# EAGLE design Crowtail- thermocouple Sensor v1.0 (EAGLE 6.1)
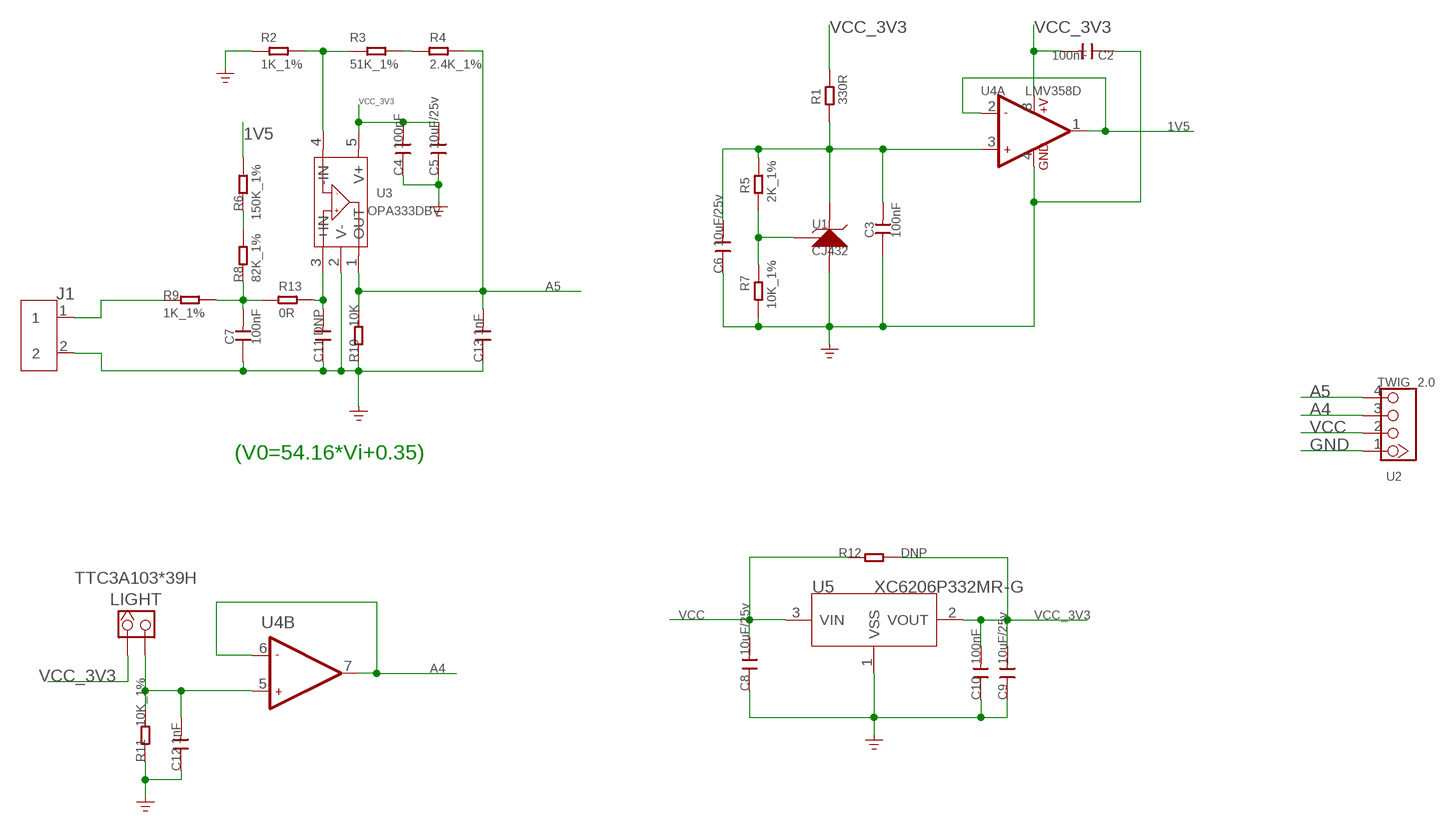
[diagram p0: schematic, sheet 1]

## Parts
C2  100nF  C-0603  [C0603]
C3  100nF  C-0603  [C0603]
C4  100nF  C-0603  [C0603]
C5  10uF/25v  C-0805  [C0805]
C6  10uF/25v  C-0805  [C0805]
C7  100nF  C-0603  [C0603]
C8  10uF/25v  C-0805  [C0805]
C9  10uF/25v  C-0805  [C0805]
C10  100nF  C-0603  [C0603]
C11  DNP  C-0603  [C0603]
C12  1nF  C-0603  [C0603]
C13  1nF  C-0603  [C0603]
J1  SCREW-TERMINAL-2P'3.5'  [2P-3.5]
LIGHT  TTC3A103*39H  HEADER_1X2_2.54  [CK_1*2]
R1  330R  R-0603  [R0603]
R2  1K_1%  R-0603  [R0603]
R3  51K_1%  R-0603  [R0603]
R4  2.4K_1%  R-0603  [R0603]
R5  2K_1%  R-0603  [R0603]
R6  150K_1%  R-0603  [R0603]
R7  10K_1%  R-0603  [R0603]
R8  82K_1%  R-0603  [R0603]
R9  1K_1%  R-0603  [R0603]
R10  10K  R-0603  [R0603]
R11  10K_1%  R-0603  [R0603]
R12  DNP  R-0603  [R0603]
R13  0R  R-0603  [R0603]
U1  CJ432  REFERENCE-SOURCE  [SOT23]
U2  TWIG_2.0  [2.0_1X4]
U3  OPA333DBV  [SOT23-5]
U4  LMV358D  [SO08]
U5  XC6206P332MR-G  XC6206MR  [SOT23]

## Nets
1V5: R6.2 U4.1(A:OUT1) U4.2(A:-IN1)
A4: U2.3 U4.6(B:-IN2) U4.7(B:OUT2)
A5: C13.2 R4.1 R10.2 U2.4 U3.1(OUT)
GND: C2.1 C3.1 C4.1 C5.1 C6.1 C7.1 C8.1 C9.1 C10.1 C11.1 C12.1 C13.1 J1.2 R2.2 R7.2 R10.1 R11.1 U1.3(A) U2.1 U3.2(V-) U4.4(A:GND) U5.1(VSS)
N$1: C7.2 R8.1 R9.2 R13.2
N$2: R2.1 R3.2 U3.4(-IN)
N$3: J1.1 R9.1
N$4: R3.1 R4.2
N$5: C12.2 LIGHT.2 R11.2 U4.5(B:+IN2)
N$6: R6.1 R8.2
N$7: C11.2 R13.1 U3.3(+IN)
N$22: R5.2 R7.1 U1.1(R)
VCC: C8.2 R12.1 U2.2 U5.3(VIN)
VCC_3V3: C2.2 C4.2 C5.2 C9.2 C10.2 LIGHT.1 R1.1 R12.2 U3.5(V+) U4.8(A:+V) U5.2(VOUT)
VREF: C3.2 C6.2 R1.2 R5.1 U1.2(K) U4.3(A:+IN1)

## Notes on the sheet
- (V0=54.16*Vi+0.35)

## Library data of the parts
C2-C13 = Discrete:C*: Ceramic Capacitors
J1 = Connector :SCREW-TERMINAL-2P
LIGHT = CONNECTER:HEADER_1X2
R1-R13 = Discrete:R*
U1 = For_Test_Albert_v6:REFERENCE-SOURCE: CJ432,AZ432 or other Adjustable Reference Source
U2 = CONNECTER:TWIG_2.0
U3 = IC:OPA333: 1.8V,Micro power CMOS oprational amplifiers Zero-Drift Series http://www.ti.com.cn/cn/lit/ds/symlink/opa333.pdf
U4 = IC:LMV358: General purpose LOW Voltage, Rail-to-Rail Output Amplifiers http://www.fairchildsemi.com/ds/LM/LMV358.pdf
U5 = IC:XC6206: LOW ESR Cap.Compatible Positive Voltage Regulators

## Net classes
0 default: width 0.152 mm, drill 0.305 mm, clearance 0.152 mm
1 power: width 0.61 mm, drill 0.406 mm, clearance 0.203 mm
2 gnd: width 0.305 mm, drill 0.559 mm, clearance 0.254 mm
3 usbvcc: width 0.508 mm, drill 0.61 mm, clearance 0.254 mm

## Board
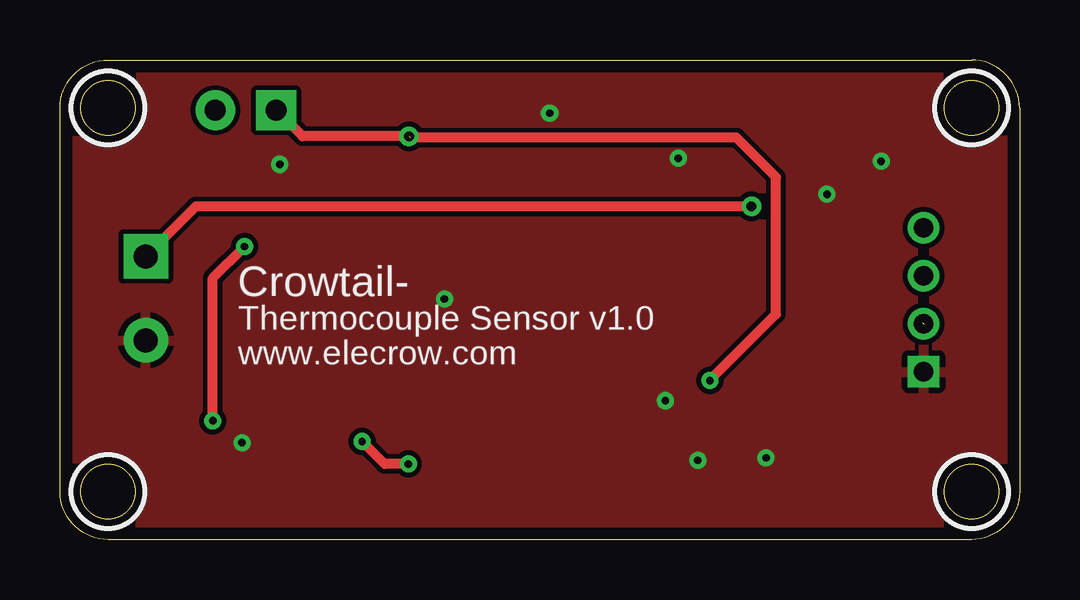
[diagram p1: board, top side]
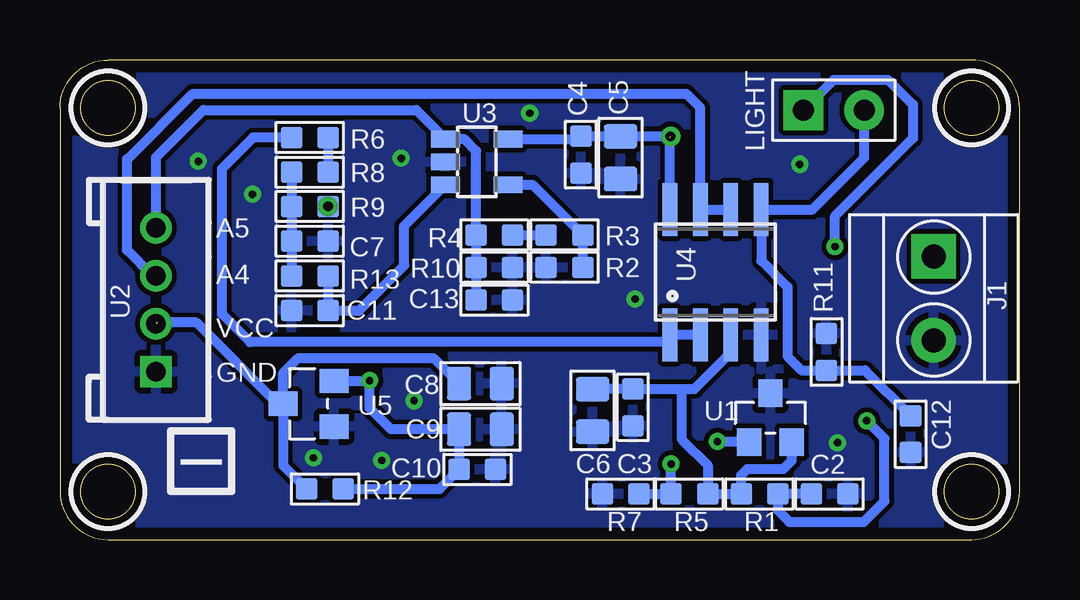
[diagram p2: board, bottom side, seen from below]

Size 40 x 20 mm. Coordinates in mm from the lower left corner, seen from the top.
Outline: 40,18 40,2 arc-90 38,0 2,0 arc-90 0,2 0,18 arc-90 2,20 38,20 arc-90 40,18
Outline: circle at 38,18 radius 1.14
Outline: circle at 38,2 radius 1.14
Outline: circle at 2,18 radius 1.14
Outline: circle at 2,2 radius 1.14
Copper layers (1*16): Top 0.035mm / dielectric 1.5mm / Bottom 0.035mm
Design rules: minimum track width 10mil, minimum drill 12mil, track to track 8mil, track to pad 8mil, pad to pad 8mil, via to via 8mil, smd to smd 0mil, copper to edge 20mil, drill to drill 8mil, minimum pad ring 10mil, minimum via ring 8mil, stop-mask expansion 2mil, vias tented up to drill 100mil, thermal gap 10mil
tRestrict: area 36.5,16.5 to 39.5,19.5; area 36.5,0.5 to 39.5,3.5; area 0.5,16.5 to 3.5,19.5; area 0.5,0.5 to 3.5,3.5
bRestrict: area 36.5,16.5 to 39.5,19.5; area 36.5,0.5 to 39.5,3.5; area 0.5,16.5 to 3.5,19.5; area 0.5,0.5 to 3.5,3.5

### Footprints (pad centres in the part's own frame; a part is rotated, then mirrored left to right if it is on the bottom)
C0603 = smd 0.889 x 0.889: 1 -0.762,0; 2 0.762,0
C0805 = smd 1.016 x 1.397: 1 -0.889,0; 2 0.889,0
2P-3.5 = drill 1 pad 1.85 square: 1 -1.75,0 | drill 1 pad 1.85: 2 1.75,0
CK_1*2 = drill 0.889 pad 1.651 square: 1 0,1.27 | drill 0.889 pad 1.651: 2 0,-1.27
R0603 = smd 0.889 x 0.889: 1 -0.762,0; 2 0.762,0
SOT23 = smd 1.016 x 1.143: 1 -0.889,-1.016; 2 0.889,-1.016; 3 0,1.016
2.0_1X4 = drill 0.8 pad 1.27 square: 1 -3,0 | drill 0.8 pad 1.27: 2 -1,0; 3 1,0; 4 3,0
SOT23-5 = smd 0.69 x 1.2: 1 -0.95,-1.3; 2 0,-1.3; 3 0.95,-1.3; 4 0.95,1.3; 5 -0.95,1.3
SO08 = smd 0.61 x 2.21: 1 -1.905,-2.616; 2 -0.635,-2.616; 3 0.635,-2.616; 4 1.905,-2.616; 5 1.905,2.616; 6 0.635,2.616; 7 -0.635,2.616; 8 -1.905,2.616
SOT23' = smd 1.016 x 1.2: 1 -0.95,-1.06; 2 0.95,-1.06; 3 0,1.06

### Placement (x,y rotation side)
C2  7.92,1.91 180 bottom
C3  16.12,5.51 90 bottom
C4  18.28,16.05 90 bottom
C5  16.63,15.93 90 bottom
C6  17.8,5.38 90 bottom
C7  29.59,12.45 180 bottom
C8  22.47,6.5 180 bottom
C9  22.47,4.6 180 bottom
C10  22.6,2.92 180 bottom
C11  29.59,9.55 0 bottom
C12  4.54,4.39 90 bottom
C13  21.89,9.98 180 bottom
J1  3.58,10.06 270 bottom
LIGHT  7.74,17.91 90 bottom
R1  10.84,1.91 180 bottom
R2  18.97,11.35 180 bottom
R3  18.97,12.7 0 bottom
R4  21.89,12.7 0 bottom
R5  13.76,1.91 180 bottom
R6  29.59,16.76 180 bottom
R7  16.63,1.91 180 bottom
R8  29.59,15.32 0 bottom
R9  29.59,13.89 180 bottom
R10  21.89,11.35 180 bottom
R11  8.05,7.82 270 bottom
R12  28.95,2.11 0 bottom
R13  29.59,11 180 bottom
U1  10.38,5.08 0 bottom
U2  36,10 90 bottom
U3  22.63,15.75 270 bottom
U4  12.67,11.15 0 bottom
U5  XC6206P332MR-G  [SOT23']  29.64,5.66 90 bottom

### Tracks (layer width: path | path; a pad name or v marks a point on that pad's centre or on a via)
1V5
  Bottom 0.406: R6.2 31.95,16.76 33.24,15.47 33.24,9.4 32.08,8.23 14.55,8.23 14.55,8.53 U4.1 U4.2
A4
  Bottom 0.406: U2.3 36.14,11 37.21,12.06 37.21,15.88 37.18,15.88 34.46,18.59 13.89,18.59 13.3,18.01 U4.7 U4.6
A5
  Bottom 0.406: U2.4 36,15.94 34.03,17.91 25.14,17.91 U3.1 23.92,16.69 23.13,16.69 22.65,16.2 R4.1 R10.2 C13.2
GND  (via drill 0.3)
  other vias: 26.59,3.3 29.43,3.4 34.23,15.77 25.78,15.9 20.42,17.78 31.97,14.4 7.59,4.04 16.02,10.03 9.16,15.65 25.24,5.79
  pour Bottom: 40,20.32 -0.64,20.32 -0.64,0 40,0
  pour Top: 40,20.32 -0.64,20.32 -0.64,0 40,0
N$1
  Bottom 0.406: R8.1 R9.2 C7.2 R13.2
N$2
  Bottom 0.406: R2.1 R3.2 20.3,14.8 U3.4
N$3  (via drill 0.41)
  Top 0.406: R9.1 5.66,13.89 J1.1
  other vias: 28.82,13.89
N$4
  Bottom 0.406: R4.2 R3.1
N$5
  Bottom 0.406: C12.2 6.45,7.06 R11.2 9.09,7.06 9.67,7.64 9.67,10.54 10.77,11.63 U4.5 8.63,13.77 6.47,15.93 LIGHT.2
N$6
  Bottom 0.406: 28.85,15.34 R8.2 R6.1
N$7
  Bottom 0.406: R13.1 C11.2 27.53,9.55 25.65,11.43 25.65,13.07 U3.3
N$22  (via drill 0.3)
  Top 0.406: v14.52,3.15 13.53,3.15 v12.59,4.09
  Bottom 0.406: R7.1 R5.2 v14.52,3.15 | v12.59,4.09 11.3,4.09 U1.1
VCC  (1 unrouted)
  Bottom 0.406: U5.3 30.93,5.66 34.31,9.04 35.96,9.04 | 29.71,2.01 R12.1 | R12.1 29.69,2.13 | R12.1 29.69,2.11 | R12.1 29.76,2.11 | U5.3 30.7,6.94 30.07,7.57 24.43,7.57 C8.2 | U5.3 30.7,3.09 R12.1
VCC_3V3  (via drill 0.3, 0.41)  (2 unrouted)
  Top 0.406: v14.55,16.82 10.1,16.82 LIGHT.1 | v6.37,4.95 6.37,10.9 v7.69,12.22 | 27.07,6.63 v27.1,6.63 27.1,6.65 29.84,9.4 29.84,15.11 28.19,16.76 14.61,16.76
  Bottom 0.406: U3.5 18.4,16.7 C4.2 C5.2 v14.55,16.82 | U4.8 14.57,16.79 14.52,16.84 | C2.2 R1.1 10.08,1.22 9.6,0.74 6.5,0.74 5.63,1.6 5.63,4.22 v6.37,4.95 | R12.2 24.18,2.11 C10.2 C9.2 26.21,4.6 27.1,5.49 v27.1,6.63 27.11,6.61 U5.2 | v7.69,12.22 7.69,13.49 4.44,16.74 4.44,18.14 5.48,19.18 7.74,19.18 LIGHT.1
VREF
  Bottom 0.406: C6.2 C3.2 14.14,6.27 | U1.2 9.49,3.3 9.85,2.95 11.35,2.95 11.6,2.69 R1.2 R5.1 13,3.1 14.07,4.17 14.07,6.2 14.14,6.27 | 14.14,6.27 13.56,6.27 12.04,7.8 | U4.3 12.04,7.8 | 12.04,7.8 12.01,7.82

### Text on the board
tPlace: Crowtail- | Thermocouple Sensor v1.0 | www.elecrow.com
bPlace: A5 | A4 | VCC | GND | I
